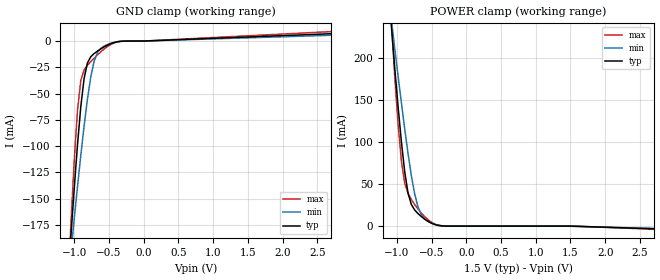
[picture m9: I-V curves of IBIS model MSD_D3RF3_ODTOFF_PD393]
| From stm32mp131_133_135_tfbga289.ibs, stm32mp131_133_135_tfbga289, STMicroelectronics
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[Model] MSD_D3RF3_ODTOFF_PD393
Model_type   Input
C_comp 2.355pF   2.274pF   2.477pF
Vinh = 925.000mV
Vinl = 575.000mV
[Temperature Range]   25.000   125.000   -40.000
[Voltage Range]   1.500V   1.425V   1.575V
[GND Clamp Reference]   0.00V   0.00V   0.00V
[POWER Clamp Reference]   1.500V   1.425V   1.575V
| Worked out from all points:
|   GND clamp passes 1 mA (typ) near -0.40 V on its own axis
|   POWER clamp passes 1 mA (typ) near -0.41 V on its own axis
[GND Clamp]
-1.48V    -635.3mA   -502.4mA   -842mA
-1.098V   -233.6mA   -234.2mA   -242.6mA
-1.05V    -186.1mA   -201.7mA   -175mA
-1.002V   -140.8mA   -169.7mA   -114.2mA
-954.6mV  -98.69mA   -138.6mA   -65.85mA
-906.8mV  -62.35mA   -108.7mA   -37.41mA
-859.1mV  -35.44mA   -80.64mA   -27.36mA
-811.4mV  -20.83mA   -55.33mA   -23.06mA
-715.9mV  -11.95mA   -19.41mA   -16.37mA
-572.7mV  -5.634mA   -4.787mA   -7.708mA
-334.1mV  -246.5uA   -315uA     -249.5uA
2.959V    7.651mA    6.016mA    9.859mA
[Power Clamp]
-1.459V   642mA      516.3mA    839.7mA
-1.077V   236mA      244.2mA    241.6mA
-1.03V    187.9mA    211.1mA    177.2mA
-981.8mV  141.9mA    178.4mA    120.7mA
-934.1mV  99.9mA     146.3mA    76.89mA
-886.4mV  64.44mA    115.4mA    50.79mA
-838.6mV  39.16mA    86.2mA     38.75mA
-743.2mV  19.18mA    38.31mA    25.69mA
-647.7mV  11.4mA     13.59mA    15.54mA
-552.3mV  5.729mA    5.637mA    7.687mA
-313.6mV  95.81uA    225.6uA    111.4uA
2.98V     -3.895mA   -3.261mA   -4.74mA
